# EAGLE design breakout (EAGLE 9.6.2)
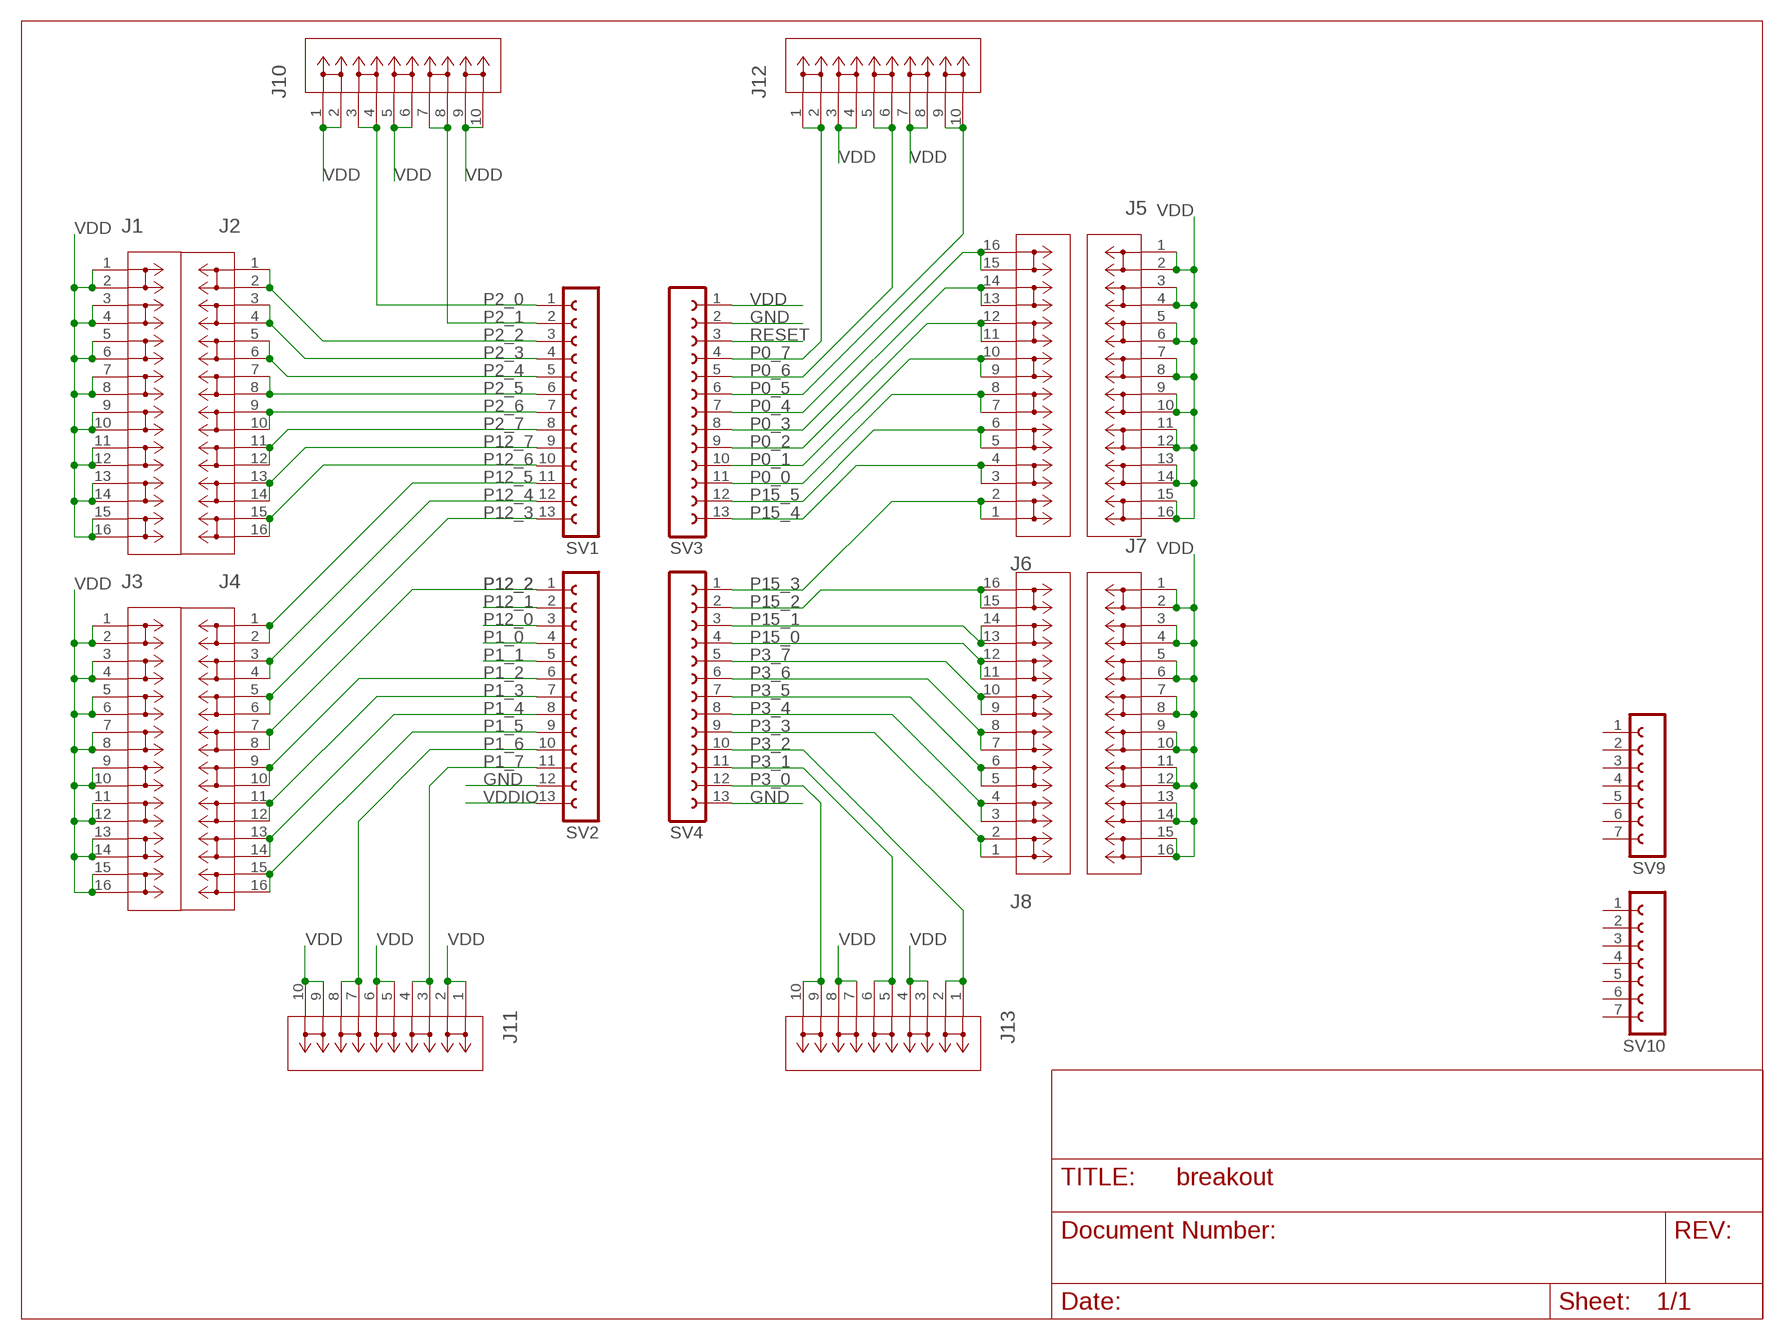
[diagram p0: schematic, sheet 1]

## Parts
J1  2601-3108CONN8_2601-3108_WAG  [CONN8_2601-3108_WAG]
J2  2601-3108CONN8_2601-3108_WAG  [CONN8_2601-3108_WAG]
J3  2601-3108CONN8_2601-3108_WAG  [CONN8_2601-3108_WAG]
J4  2601-3108CONN8_2601-3108_WAG  [CONN8_2601-3108_WAG]
J5  2601-3108CONN8_2601-3108_WAG  [CONN8_2601-3108_WAG]
J6  2601-3108CONN8_2601-3108_WAG  [CONN8_2601-3108_WAG]
J7  2601-3108CONN8_2601-3108_WAG  [CONN8_2601-3108_WAG]
J8  2601-3108CONN8_2601-3108_WAG  [CONN8_2601-3108_WAG]
J10  2601-3105CONN5_2601-3105_WAG  [CONN5_2601-3105_WAG]
J11  2601-3105CONN5_2601-3105_WAG  [CONN5_2601-3105_WAG]
J12  2601-3105CONN5_2601-3105_WAG  [CONN5_2601-3105_WAG]
J13  2601-3105CONN5_2601-3105_WAG  [CONN5_2601-3105_WAG]
SV1  FE13-1  [FE13]
SV2  FE13-1  [FE13]
SV3  FE13-1  [FE13]
SV4  FE13-1  [FE13]
SV9  FE07-1  [FE07]
SV10  FE07-1  [FE07]

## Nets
GND: SV2.12 SV3.2 SV4.13
P0_0: J6.7(4_1) J6.8(4_2) SV3.11
P0_1: J6.9(5_1) J6.10(5_2) SV3.10
P0_2: J6.11(6_1) J6.12(6_2) SV3.9
P0_3: J6.13(7_1) J6.14(7_2) SV3.8
P0_4: J6.15(8_1) J6.16(8_2) SV3.7
P0_5: J12.9(5_1) J12.10(5_2) SV3.6
P0_6: J12.5(3_1) J12.6(3_2) SV3.5
P0_7: J12.1(1_1) J12.2(1_2) SV3.4
P1_0: SV2.4
P1_1: SV2.5
P1_2: J4.9(5_1) J4.10(5_2) SV2.6
P1_3: J4.11(6_1) J4.12(6_2) SV2.7
P1_4: J4.13(7_1) J4.14(7_2) SV2.8
P1_5: J4.15(8_1) J4.16(8_2) SV2.9
P1_6: J11.7(4_1) J11.8(4_2) SV2.10
P1_7: J11.3(2_1) J11.4(2_2) SV2.11
P2_0: J10.3(2_1) J10.4(2_2) SV1.1
P2_1: J10.7(4_1) J10.8(4_2) SV1.2
P2_2: J2.1(1_1) J2.2(1_2) SV1.3
P2_3: J2.3(2_1) J2.4(2_2) SV1.4
P2_4: J2.5(3_1) J2.6(3_2) SV1.5
P2_5: J2.7(4_1) J2.8(4_2) SV1.6
P2_6: J2.9(5_1) J2.10(5_2) SV1.7
P2_7: J2.11(6_1) J2.12(6_2) SV1.8
P3_0: J13.9(5_1) J13.10(5_2) SV4.12
P3_1: J13.5(3_1) J13.6(3_2) SV4.11
P3_2: J13.1(1_1) J13.2(1_2) SV4.10
P3_3: J8.1(1_1) J8.2(1_2) SV4.9
P3_4: J8.3(2_1) J8.4(2_2) SV4.8
P3_5: J8.5(3_1) J8.6(3_2) SV4.7
P3_6: J8.7(4_1) J8.8(4_2) SV4.6
P3_7: J8.9(5_1) J8.10(5_2) SV4.5
P12_0: SV2.3
P12_1: SV2.2
P12_2: J4.7(4_1) J4.8(4_2) SV2.1
P12_3: J4.5(3_1) J4.6(3_2) SV1.13
P12_4: J4.3(2_1) J4.4(2_2) SV1.12
P12_5: J4.1(1_1) J4.2(1_2) SV1.11
P12_6: J2.15(8_1) J2.16(8_2) SV1.10
P12_7: J2.13(7_1) J2.14(7_2) SV1.9
P15_0: J8.11(6_1) J8.12(6_2) SV4.4
P15_1: J8.13(7_1) J8.14(7_2) SV4.3
P15_2: J8.15(8_1) J8.16(8_2) SV4.2
P15_3: J6.1(1_1) J6.2(1_2) SV4.1
P15_4: J6.3(2_1) J6.4(2_2) SV3.13
P15_5: J6.5(3_1) J6.6(3_2) SV3.12
RESET: SV3.3
VDD: J1.1(1_1) J1.2(1_2) J1.3(2_1) J1.4(2_2) J1.5(3_1) J1.6(3_2) J1.7(4_1) J1.8(4_2) J1.9(5_1) J1.10(5_2) J1.11(6_1) J1.12(6_2) J1.13(7_1) J1.14(7_2) J1.15(8_1) J1.16(8_2) J3.1(1_1) J3.2(1_2) J3.3(2_1) J3.4(2_2) J3.5(3_1) J3.6(3_2) J3.7(4_1) J3.8(4_2) J3.9(5_1) J3.10(5_2) J3.11(6_1) J3.12(6_2) J3.13(7_1) J3.14(7_2) J3.15(8_1) J3.16(8_2) J5.1(1_1) J5.2(1_2) J5.3(2_1) J5.4(2_2) J5.5(3_1) J5.6(3_2) J5.7(4_1) J5.8(4_2) J5.9(5_1) J5.10(5_2) J5.11(6_1) J5.12(6_2) J5.13(7_1) J5.14(7_2) J5.15(8_1) J5.16(8_2) J7.1(1_1) J7.2(1_2) J7.3(2_1) J7.4(2_2) J7.5(3_1) J7.6(3_2) J7.7(4_1) J7.8(4_2) J7.9(5_1) J7.10(5_2) J7.11(6_1) J7.12(6_2) J7.13(7_1) J7.14(7_2) J7.15(8_1) J7.16(8_2) J10.1(1_1) J10.2(1_2) J10.5(3_1) J10.6(3_2) J10.9(5_1) J10.10(5_2) J11.1(1_1) J11.2(1_2) J11.5(3_1) J11.6(3_2) J11.9(5_1) J11.10(5_2) J12.3(2_1) J12.4(2_2) J12.7(4_1) J12.8(4_2) J13.3(2_1) J13.4(2_2) J13.7(4_1) J13.8(4_2) SV3.1
VDDIO: SV2.13
Unconnected: SV9.1 SV9.2 SV9.3 SV9.4 SV9.5 SV9.6 SV9.7 SV10.1 SV10.2 SV10.3 SV10.4 SV10.5 SV10.6 SV10.7

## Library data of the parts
J1-J8 = 2025-03-15_17-36-39_Library:2601-3108; COPYRIGHT: Copyright (C) 2025 Ultra Librarian. All rights reserved.; MANUFACTURER_PART_NUMBER: 2601-3108; MFR_NAME: Wago
J10-J13 = 2025-04-13_04-35-33_Library:2601-3105; COPYRIGHT: Copyright (C) 2025 Ultra Librarian. All rights reserved.; MANUFACTURER_PART_NUMBER: 2601-3105; MFR_NAME: Wago
SV1-SV4 = con-lsta:FE13-1: FEMALE HEADER; OC_FARNELL: unknown; OC_NEWARK: unknown
SV9 SV10 = con-lsta:FE07-1: FEMALE HEADER; OC_FARNELL: unknown; OC_NEWARK: unknown

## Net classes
0 default: width 0.254 mm, clearance 0.254 mm

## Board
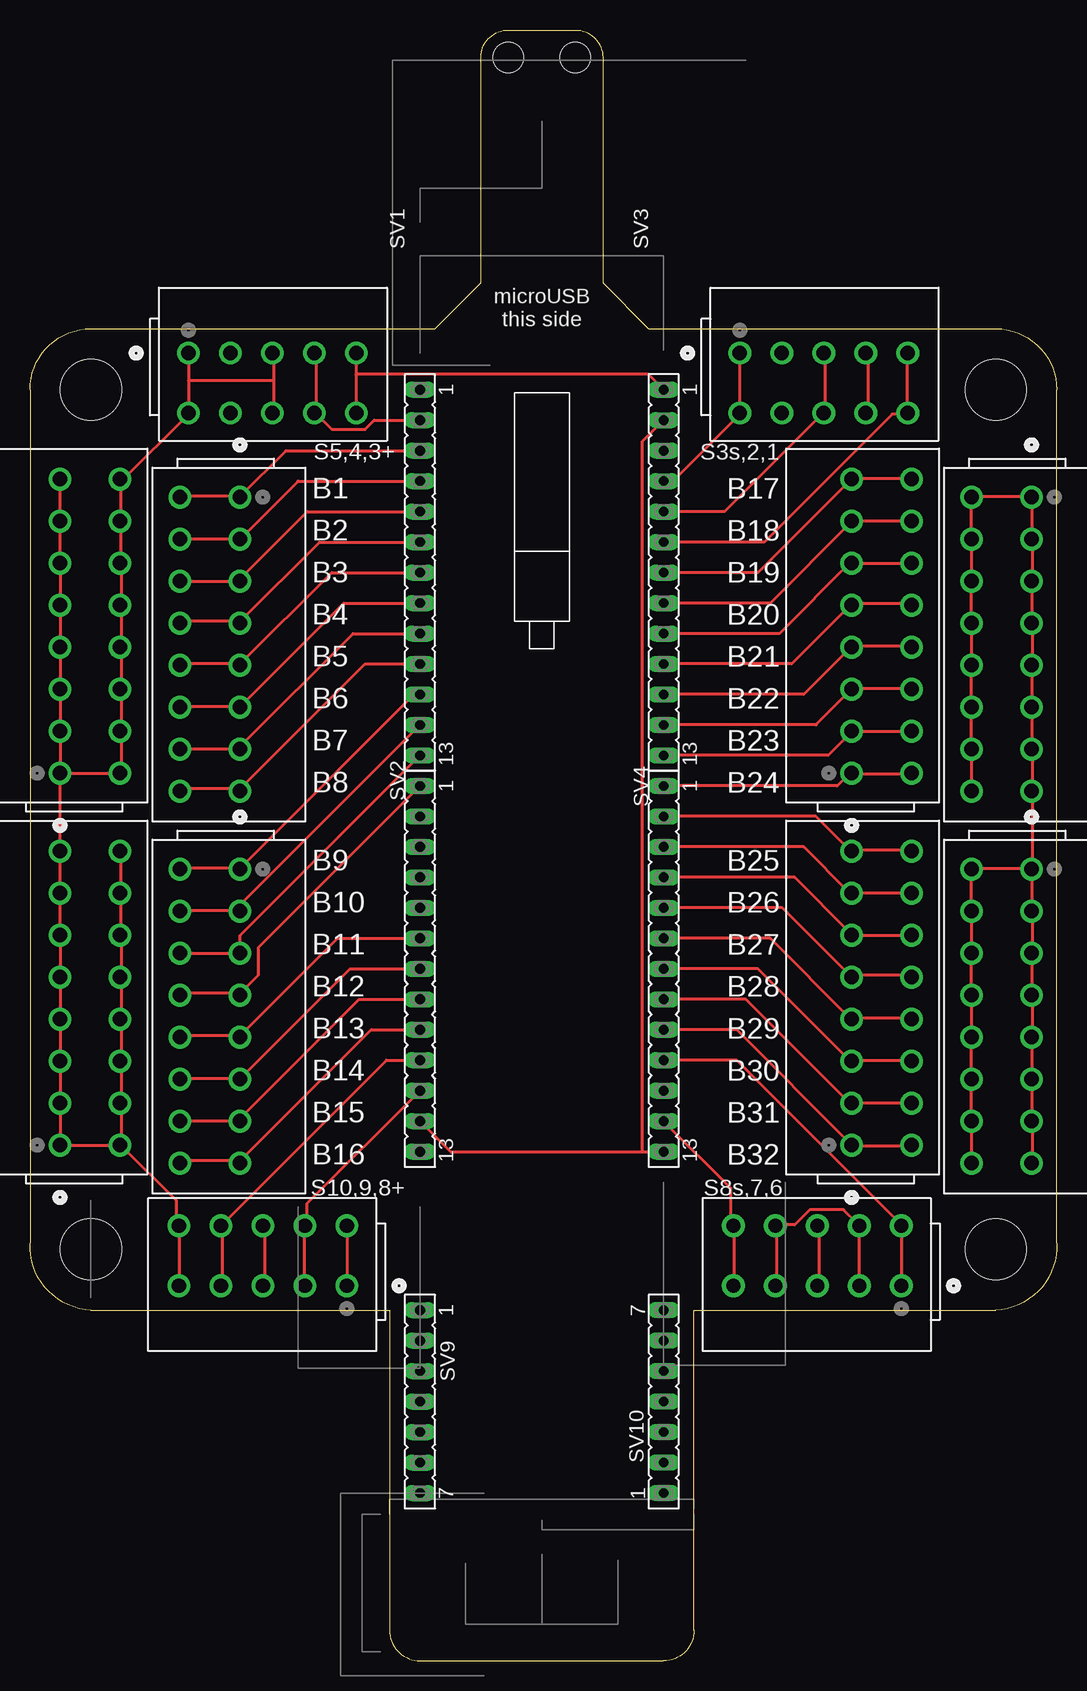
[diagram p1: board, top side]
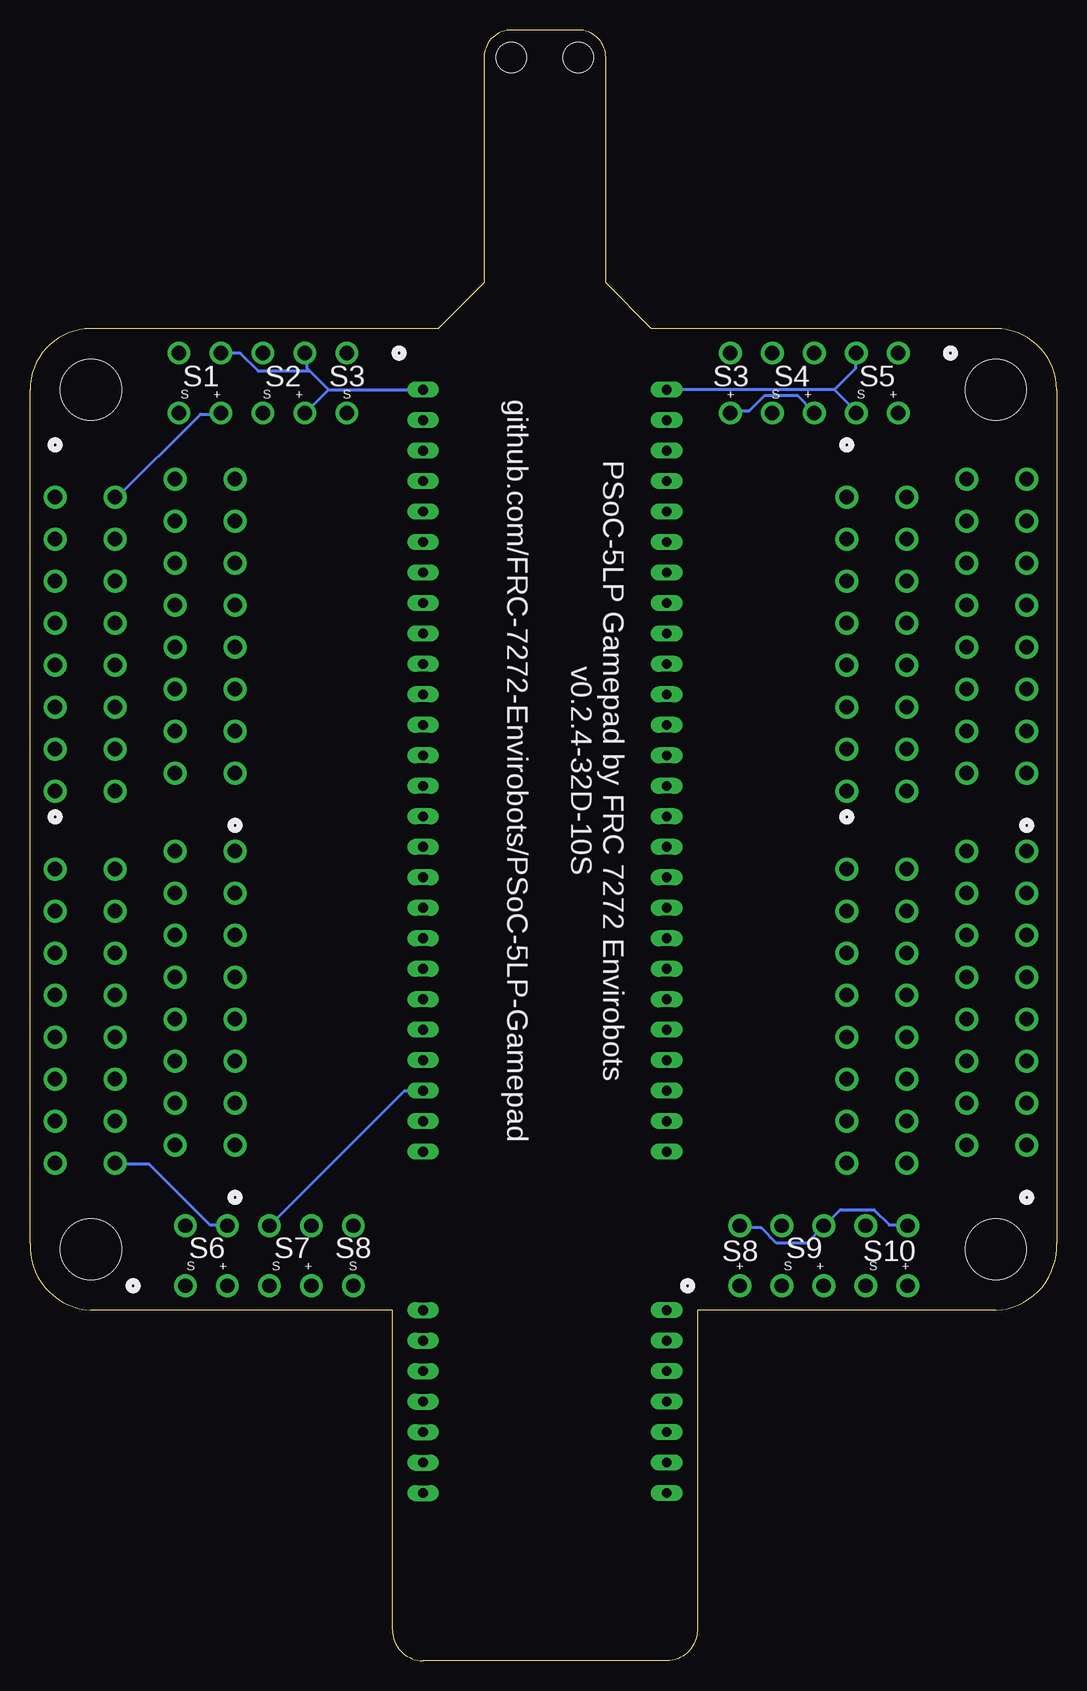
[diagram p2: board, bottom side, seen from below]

Size 85.6 x 135.89 mm. Coordinates in mm from the lower left corner, seen from the top.
Outline: 80.52,111 81.03,111
Outline: 80.52,111 arc-90 85.6,105.92 85.6,34.8 arc-90 80.52,29.21 55.37,29.21 55.37,2.54 arc-90 52.83,0 32.51,0 arc-90 29.97,2.54 29.97,29.21 5.08,29.21 arc-90 0,34.8 0,105.92 arc-90 5.08,111 33.78,111 37.59,114.81 37.59,133.6 arc-90 39.88,135.89 45.47,135.89 arc-90 47.75,133.6 47.75,114.81 51.56,111 80.52,111
Copper layers (1*16): Top 0.035mm / dielectric 1.5mm / Bottom 0.035mm
Design rules "default": minimum track width 6mil, minimum drill 0.35mm, track to track 6mil, track to pad 6mil, pad to pad 6mil, via to via 6mil, smd to smd 6mil, copper to edge 40mil, drill to drill 6mil, minimum pad ring 10mil, minimum via ring 8mil, stop-mask expansion 4mil, vias tented up to drill 0mil, thermal gap 10mil
Holes 2.54 mm at 39.88,133.6 45.47,133.6
Holes 5.08 mm at 5.08,105.92 80.52,105.92 5.08,34.29 80.52,34.29

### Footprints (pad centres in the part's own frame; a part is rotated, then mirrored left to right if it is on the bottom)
CONN8_2601-3108_WAG = drill 1.2 pad 1.9: 1 0,0; 2 0,-5; 3 3.5,0; 4 3.5,-5; 5 7,0; 6 7,-5; 7 10.5,0; 8 10.5,-5; 9 14,0; 10 14,-5; 11 17.5,0; 12 17.5,-5; 13 21,0; 14 21,-5; 15 24.5,0; 16 24.5,-5
CONN5_2601-3105_WAG = drill 1.2 pad 1.9: 1 0,0; 2 0,-5; 3 3.5,0; 4 3.5,-5; 5 7,0; 6 7,-5; 7 10.5,0; 8 10.5,-5; 9 14,0; 10 14,-5
FE13 = drill 0.813 long: 1 -15.24,0; 2 -12.7,0; 3 -10.16,0; 4 -7.62,0; 5 -5.08,0; 6 -2.54,0; 7 0,0; 8 2.54,0; 9 5.08,0; 10 7.62,0; 11 10.16,0; 12 12.7,0; 13 15.24,0
FE07 = drill 0.813 long: 1 -7.62,0; 2 -5.08,0; 3 -2.54,0; 4 0,0; 5 2.54,0; 6 5.08,0; 7 7.62,0

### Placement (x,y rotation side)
J1  2.5,73.96 90 top
J2  17.5,96.96 270 top
J3  2.5,42.96 90 top
J4  17.5,65.96 270 top
J5  83.5,96.96 270 top
J6  68.5,73.96 90 top
J7  83.5,65.96 270 top
J8  68.5,42.96 90 top
J10  13.21,108.97 0 top
J11  26.42,31.24 180 top
J12  59.18,108.97 0 top
J13  72.64,31.24 180 top
SV1  32.51,90.68 270 top
SV2  32.51,57.66 270 top
SV3  52.83,90.68 270 top
SV4  52.83,57.66 270 top
SV9  32.51,21.59 270 top
SV10  52.83,21.59 90 top

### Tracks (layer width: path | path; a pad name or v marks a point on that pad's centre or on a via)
GND
  Top 0.254: 51.05,42.42 35.05,42.42 SV2.12 | 51.05,42.42 SV4.13 | SV3.2 51.05,101.6 51.05,42.42
P0_0
  Top 0.254: SV3.11 64.52,80.52 68.33,84.33 J6.7 68.58,84.58 73.41,84.58 J6.8
P0_1
  Top 0.254: SV3.10 63.5,83.06 68.33,87.88 J6.9 68.58,88.14 73.41,88.14 J6.10
P0_2
  Top 0.254: SV3.9 62.48,85.6 68.33,91.44 J6.11 68.58,91.44 73.41,91.44 J6.12
P0_3
  Top 0.254: SV3.8 61.72,88.14 68.33,94.74 J6.13 68.58,95 73.41,95 J6.14
P0_4
  Top 0.254: SV3.7 60.71,90.68 68.33,98.3 J6.15 68.58,98.55 73.41,98.55 J6.16
P0_5
  Top 0.254: SV3.6 61.21,93.22 71.88,103.89 73.15,103.89 J12.10 73.15,104.14 73.15,108.97 J12.9
P0_6
  Top 0.254: SV3.5 57.91,95.76 66.04,103.89 J12.6 66.29,104.14 66.29,108.97 J12.5
P0_7
  Top 0.254: SV3.4 53.59,98.3 59.18,103.89 J12.2 J12.1
P1_2
  Top 0.254: SV2.6 25.65,60.2 17.53,52.07 J4.9 17.27,52.07 12.7,52.07 J4.10
P1_3
  Top 0.254: SV2.7 26.67,57.66 17.53,48.51 J4.11 17.27,48.51 12.7,48.51 J4.12
P1_4
  Top 0.254: SV2.8 27.43,55.12 17.53,45.21 J4.13 17.27,44.96 12.7,44.96 J4.14
P1_5
  Top 0.254: SV2.9 28.45,52.58 17.53,41.66 J4.15 17.27,41.66 12.7,41.66 J4.16
P1_6
  Top 0.254: SV2.10 29.72,50.04 16,36.32 J11.8 16,36.07 16,31.24 J11.7
P1_7
  Top 0.254: SV2.11 23.11,38.1 23.11,36.32 J11.4 22.86,36.07 22.86,31.24 J11.3
P2_0
  Bottom 0.254: 18.54,105.92 SV1.1 | 18.54,105.92 16.76,104.14 J10.4 | 18.54,105.92 16.76,107.7 16.76,108.97 J10.3
P2_1
  Top 0.254: SV1.2 28.7,103.38 27.94,102.62 25.15,102.62 23.88,103.89 J10.8 23.88,104.14 23.88,108.97 J10.7
P2_2
  Top 0.254: SV1.3 21.34,100.84 17.53,97.03 J2.1 17.27,97.03 12.7,97.03 J2.2
P2_3
  Top 0.254: SV1.4 22.35,98.3 17.53,93.47 J2.3 17.27,93.47 12.7,93.47 J2.4
P2_4
  Top 0.254: SV1.5 23.11,95.76 17.53,90.17 J2.5 17.27,89.92 12.7,89.92 J2.6
P2_5
  Top 0.254: SV1.6 24.13,93.22 17.53,86.61 J2.7 17.27,86.61 12.7,86.61 J2.8
P2_6
  Top 0.254: SV1.7 25.15,90.68 17.53,83.06 J2.9 17.27,83.06 12.7,83.06 J2.10
P2_7
  Top 0.254: SV1.8 26.16,88.14 17.53,79.5 J2.11 17.27,79.5 12.7,79.5 J2.12
P3_0
  Top 0.254: SV4.12 58.42,39.37 58.42,36.32 J13.10 58.67,36.07 58.67,31.24 J13.9
P3_1
  Top 0.254: J13.5 65.79,31.24 65.79,36.07 J13.6
  Bottom 0.254: SV4.11 54.36,47.5 65.53,36.32 J13.6
P3_2
  Top 0.254: SV4.10 58.93,50.04 72.64,36.32 J13.2 J13.1
P3_3
  Top 0.254: SV4.9 58.93,52.58 68.33,43.18 J8.1 68.58,42.93 73.41,42.93 J8.2
P3_4
  Top 0.254: SV4.8 59.69,55.12 68.33,46.48 J8.3 68.58,46.48 73.41,46.48 J8.4
P3_5
  Top 0.254: SV4.7 60.71,57.66 68.33,50.04 J8.5 68.58,50.04 73.41,50.04 J8.6
P3_6
  Top 0.254: SV4.6 61.72,60.2 68.33,53.59 J8.7 68.58,53.59 73.41,53.59 J8.8
P3_7
  Top 0.254: SV4.5 62.74,62.74 68.33,57.15 J8.9 68.58,57.15 73.41,57.15 J8.10
P12_2
  Top 0.254: SV2.1 19.05,59.44 19.05,57.15 17.53,55.63 J4.7 17.27,55.63 12.7,55.63 J4.8
P12_3
  Top 0.254: SV1.13 17.53,60.45 17.53,59.18 J4.5 17.27,58.93 12.7,58.93 J4.6
P12_4
  Top 0.254: SV1.12 17.53,62.99 17.53,62.48 J4.3 17.27,62.48 12.7,62.48 J4.4
P12_5
  Top 0.254: SV1.11 32,80.52 17.53,66.04 J4.1 17.27,66.04 12.7,66.04 J4.2
P12_6
  Top 0.254: SV1.10 27.94,83.06 17.53,72.64 J2.15 17.27,72.64 12.7,72.64 J2.16
P12_7
  Top 0.254: SV1.9 26.92,85.6 17.53,76.2 J2.13 17.27,75.95 12.7,75.95 J2.14
P15_0
  Top 0.254: SV4.4 63.75,65.28 68.33,60.71 J8.11 68.58,60.45 73.41,60.45 J8.12
P15_1
  Top 0.254: SV4.3 64.52,67.82 68.33,64.01 J8.13 68.58,64.01 73.41,64.01 J8.14
P15_2
  Top 0.254: SV4.2 65.53,70.36 68.33,67.56 J8.15 68.58,67.56 73.41,67.56 J8.16
P15_3
  Top 0.254: SV4.1 67.31,72.9 68.33,73.91 J6.1 68.58,73.91 73.41,73.91 J6.2
P15_4
  Top 0.254: SV3.13 66.55,75.44 68.33,77.22 J6.3 68.58,77.47 73.41,77.47 J6.4
P15_5
  Top 0.254: SV3.12 65.53,77.98 68.33,80.77 J6.5 68.58,81.03 73.41,81.03 J6.6
VDD
  Top 0.254: J1.15 2.54,98.3 2.54,95 J1.13 2.54,94.74 2.54,91.69 J1.11 2.54,91.44 2.54,88.14 J1.9 2.54,87.88 2.54,84.58 J1.7 2.54,84.33 2.54,81.03 J1.5 2.54,80.77 2.54,77.47 J1.3 2.54,77.22 2.54,74.17 J1.1 2.54,73.91 | 27.18,107.19 27.18,108.97 J10.9 | 27.18,107.19 27.18,104.14 J10.10 | J10.1 13.21,106.68 | 13.21,106.68 J10.2 13.21,103.89 7.62,98.3 | 20.32,106.68 20.32,108.97 J10.5 | 20.32,106.68 20.32,104.14 J10.6 | 20.32,106.68 13.21,106.68 | 7.62,98.3 7.62,95 J1.14 7.62,94.74 7.62,91.69 J1.12 7.62,91.44 7.62,88.14 J1.10 7.62,87.88 7.62,84.58 J1.8 7.62,84.33 7.62,81.03 J1.6 7.62,80.77 7.62,77.47 J1.4 7.62,77.22 7.62,74.17 J1.2 7.37,73.91 2.54,73.91 | 7.62,98.3 J1.16 | J11.2 J11.1 | J11.9 12.45,31.24 12.45,36.07 J11.10 12.19,36.32 12.19,38.35 7.62,42.93 J3.2 | J11.5 19.56,31.24 19.56,36.07 J11.6 | J3.2 7.62,43.18 7.62,46.23 J3.4 7.62,46.48 7.62,49.78 J3.6 7.62,50.04 7.62,53.34 J3.8 7.62,53.59 7.62,56.9 J3.10 7.62,57.15 7.62,60.45 J3.12 7.62,60.71 7.62,63.75 J3.14 7.62,64.01 7.62,67.31 J3.16 | J3.2 7.37,42.93 2.54,42.93 J3.1 2.54,43.18 2.54,46.23 J3.3 2.54,46.48 2.54,49.78 J3.5 2.54,50.04 2.54,53.34 J3.7 2.54,53.59 2.54,56.9 J3.9 2.54,57.15 2.54,60.45 J3.11 2.54,60.71 2.54,63.75 J3.13 2.54,64.01 2.54,67.31 J3.15 2.54,67.56 2.54,73.91 | J7.1 83.57,65.79 83.57,62.48 J7.3 83.57,62.23 83.57,59.18 J7.5 83.57,58.93 83.57,55.63 J7.7 83.57,55.37 83.57,52.07 J7.9 83.57,51.82 83.57,48.51 J7.11 83.57,48.26 83.57,45.21 J7.13 83.57,44.96 83.57,41.66 J7.15 | J13.7 62.23,31.24 62.23,36.07 J13.8 62.23,36.32 63.75,36.32 65.02,37.59 67.82,37.59 69.09,36.32 J13.4 69.09,36.07 69.09,31.24 J13.3
  Top 0.254: J7.16 78.49,41.66 78.49,44.96 J7.14 78.49,45.21 78.49,48.26 J7.12 78.49,48.51 78.49,51.82 J7.10 78.49,52.07 78.49,55.37 J7.8 78.49,55.63 78.49,58.93 J7.6 78.49,59.18 78.49,62.23 J7.4 78.49,62.48 78.49,65.79 J7.2 78.74,66.04 83.31,66.04 J7.1 | J12.8 69.85,104.14 69.85,108.97 J12.7 | J5.16 78.49,72.64 78.49,75.95 J5.14 78.49,76.2 78.49,79.25 J5.12 78.49,79.5 78.49,82.8 J5.10 78.49,83.06 78.49,86.36 J5.8 78.49,86.61 78.49,89.92 J5.6 78.49,90.17 78.49,93.22 J5.4 78.49,93.47 78.49,96.77 J5.2 78.74,97.03 83.31,97.03 J5.1 83.57,96.77 83.57,93.47 J5.3 83.57,93.22 83.57,90.17 J5.5 83.57,89.92 83.57,86.61 J5.7 83.57,86.36 83.57,83.06 J5.9 83.57,82.8 83.57,79.5 J5.11 83.57,79.25 83.57,76.2 J5.13 83.57,75.95 83.57,72.64 J5.15 83.57,72.39 83.57,66.04 J7.1 | 27.18,107.19 51.56,107.19 SV3.1
  Bottom 0.254: J10.10 27.18,104.14 25.65,104.14 24.38,105.41 21.59,105.41 20.32,104.14 J10.6 | J11.10 12.45,36.32 13.97,36.32 15.24,37.59 18.03,37.59 19.3,36.32 J11.6 19.56,36.07 20.83,34.8 23.37,34.8 24.64,36.07 26.42,36.07 J11.2 | J13.4 69.34,36.32 70.61,36.32 75.69,41.4 78.49,41.4 J7.16 | 60.71,105.92 SV3.1 | 60.71,105.92 62.48,104.14 J12.4 | 60.71,105.92 62.23,107.44 | 62.23,107.44 62.48,107.7 62.48,108.97 J12.3 | J12.7 68.07,108.97 66.55,107.44 62.23,107.44 | J12.8 69.85,103.89 71.37,103.89 78.49,96.77 J5.2

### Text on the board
tPlace: microUSB / this side | S5,4,3+ | S3s,2,1 | B1 | B17 | B2 | B18 | B3 | B19 | B4 | B20 | B5 | B21 | B6 | B22 | B7 | B23 | B8 | B24 | B9 | B25 | B10 | B26 | B11 | B27 | B12 | B28 | B13 | B29 | B14 | B30 | B15 | B31 | B16 | B32 | S10,9,8+ | S8s,7,6
bPlace: S5 | S4 | S3 | S3 | S2 | S1 | S + | S + | + | S | S + | S + | PSoC-5LP Gamepad by FRC 7272 Envirobots / v0.2.4-32D-10S / / github.com/FRC-7272-Envirobots/PSoC-5LP-Gamepad | S + | S10 | S + | S9 | + | S8 | S | S8 | S + | S7 | S + | S6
